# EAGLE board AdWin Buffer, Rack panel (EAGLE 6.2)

No outline drawn. Coordinates in mm, seen from the top.
Copper layers (1+16): Top 0.035mm / dielectric 1.5mm / Bottom 0.035mm
Design rules: minimum track width 7mil, minimum drill 20mil, track to track 7mil, track to pad 7mil, pad to pad 7mil, via to via 7mil, smd to smd 0mil, copper to edge 25mil, drill to drill 8mil, minimum pad ring 10mil, minimum via ring 8mil, stop-mask expansion 4mil, vias tented up to drill 0mil, thermal gap 10mil
Net classes: 0 default: drill 0.508 mm; 1 PowerA: width 0.406 mm, drill 0.711 mm; 2 Power clearance: width 0.406 mm, drill 0.711 mm, clearance 0.508 mm
Holes 12.7 mm at 85.16,35.18 105.48,35.18 125.8,35.18 146.12,35.18 166.44,35.18 186.76,35.18 227.4,35.18 207.08,35.18 85.16,97.41 105.48,97.41 125.8,97.41 146.12,97.41 166.44,97.41 186.76,97.41 227.4,97.41 207.08,97.41 252.8,35.18 273.12,35.18 293.44,35.18 313.76,35.18 334.08,35.18 354.4,35.18 374.72,35.18 395.04,35.18 252.8,97.41 273.12,97.41 293.44,97.41 313.76,97.41 334.08,97.41 354.4,97.41 374.72,97.41 395.04,97.41
Holes 2.92 mm at 86.43,45.97 106.75,45.97 127.07,45.97 147.39,45.97 167.71,45.97 188.03,45.97 208.35,45.97 228.67,45.97 254.07,45.97 274.39,45.97 294.71,45.97 315.03,45.97 335.35,45.97 355.67,45.97 375.99,45.97 396.31,45.97 86.43,108.2 106.75,108.2 127.07,108.2 147.39,108.2 167.71,108.2 188.03,108.2 208.35,108.2 228.67,108.2 254.07,108.2 274.39,108.2 294.71,108.2 315.03,108.2 335.35,108.2 355.67,108.2 375.99,108.2 396.31,108.2

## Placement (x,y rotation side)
U$5  [CASE:RACK,PANEL,3U]  0,0 0 top
U$19  [TITLEBLOCK_PCB]  0.64,-10.79 0 top

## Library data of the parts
U$5 U$19 = QuantumOptics

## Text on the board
Reference: 3.40 | 4.20 | 5.00 | 5.80 | 6.60 | 7.40 | 8.20 | 9.00 | 10.00 | 10.80 | 11.60 | 12.40 | 13.20 | 14.00 | 14.80 | 15.60 | 5.22 (ref) | 4.25 | 0.115" +0.003 - 0.002 | 32 places | 3.835 | 0.505" +0.005 - 0.000 | 32 places | 1.81 | 1.385 | 0" | 0" | 3.35 | 4.15 | 4.95 | 5.75 | 6.55 | 7.35 | 8.15 | 8.95 | 9.95 | 10.75 | 11.55 | 12.35 | 13.15 | 13.95 | 14.75 | 15.55 | 19 (ref)
Target: ADWin Digital Buffer | J. Thywissen Labs | A. Stummer June 2012 | F | Panel such as Hammond PBPA19005UNF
